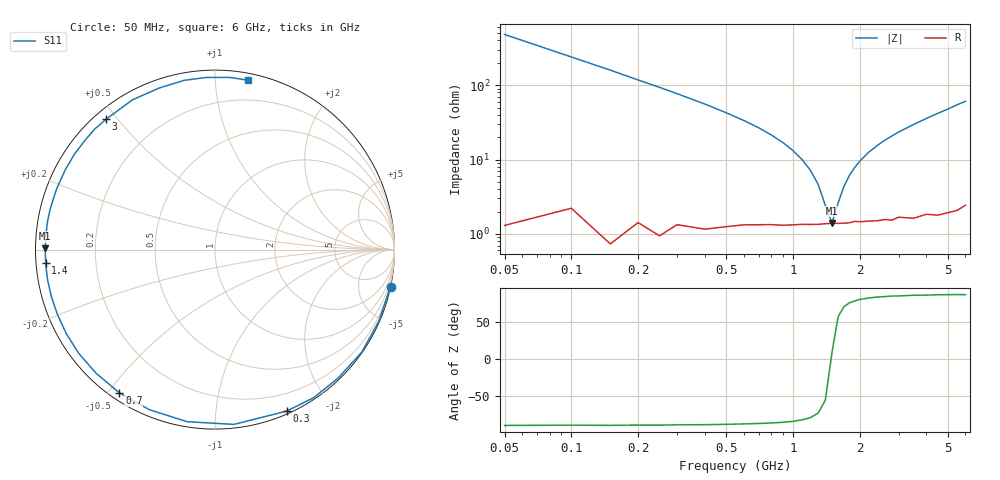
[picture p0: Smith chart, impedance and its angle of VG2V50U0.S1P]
! Infineon Technologies  Discrete & RF Semiconductors
! BB 831
! Si Tuning Diode in SOD323
! VR = 2.5 V
! S-Parameters:  July  1999
# GHz  S  MA  R  50
!  f  S11
! GHz  MAG  ANG
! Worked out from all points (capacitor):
!   34 points, 50 MHz to 6 GHz, reference 50 ohm
!   read as one part to ground: C = 6.62 pF near 50 MHz
!   lowest |Z| = 1.41 ohm at 1.5 GHz (marker M1)
!   series resonance near 1.49 GHz, so ESL is about 1.7 nH
!   S11 on the Smith chart (normalised r, x): 50 MHz: 0.03, -9.59; 300 MHz: 0.03, -1.54; 700 MHz: 0.03, -0.53; 1.4 GHz: 0.03, -0.04; 3 GHz: 0.03, +0.47; 6 GHz: 0.05, +1.21
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0.05  0.9994 -11.9
0.1  0.9963 -23.6
0.15  0.9974 -34.9
0.2  0.9913 -46.1
0.25  0.9916 -56.3
0.3  0.9843 -66.1
0.4  0.9795 -83.8
0.5  0.9714 -99.2
0.6  0.964 -112.3
0.7  0.9595 -123.7
0.8  0.9558 -133.8
0.9  0.9541 -142.6
1.1  0.9494 -157.6
1.2  0.9487 -164.0
1.4  0.9466 -175.4
1.5  0.9459 179.5
1.6  0.9461 174.9
1.8  0.9457 166.3
2  0.9452 158.8
2.4  0.9466 145.8
2.6  0.9462 140.0
3  0.9463 129.8
3.5  0.9529 118.9
4  0.9524 108.9
4.5  0.9586 100.3
5  0.9603 92.8
5.5  0.9629 85.1
6  0.9614 79.1
